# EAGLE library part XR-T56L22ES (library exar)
PCM REPEATER/RECEIVER
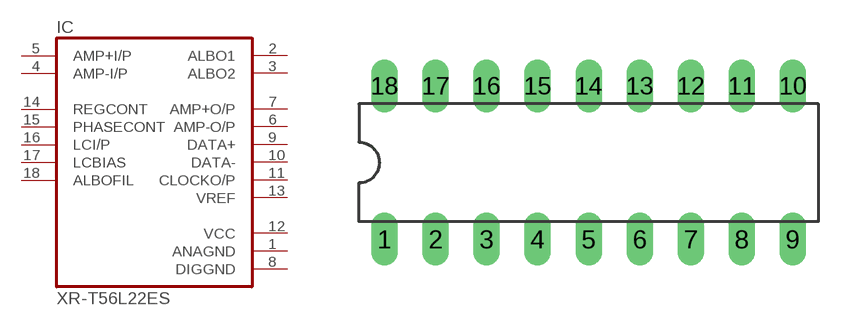
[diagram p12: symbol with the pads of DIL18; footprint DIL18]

Designator prefix IC

## XR-T56L22ES (OC_FARNELL: unknown; OC_NEWARK: unknown)  [DIL18]
1  ANAGND  pwr
2  ALBO1  out
3  ALBO2  out
4  AMP-I/P  in
5  AMP+I/P  in
6  AMP-O/P  out
7  AMP+O/P  out
8  DIGGND  pwr
9  DATA+  out
10  DATA-  out
11  CLOCKO/P  out
12  VCC  pwr
13  VREF  out
14  REGCONT  in
15  PHASECONT  in
16  LCI/P  in
17  LCBIAS  in
18  ALBOFIL  in

## Footprint DIL18 (pad centres in mm)
Dual In Line Package
drill 0.813 long: 1 -10.16,-3.81; 2 -7.62,-3.81; 3 -5.08,-3.81; 4 -2.54,-3.81; 5 0,-3.81; 6 2.54,-3.81; 7 5.08,-3.81; 8 7.62,-3.81; 9 10.16,-3.81; 10 10.16,3.81; 11 7.62,3.81; 12 5.08,3.81; 13 2.54,3.81; 14 0,3.81; 15 -2.54,3.81; 16 -5.08,3.81; 17 -7.62,3.81; 18 -10.16,3.81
